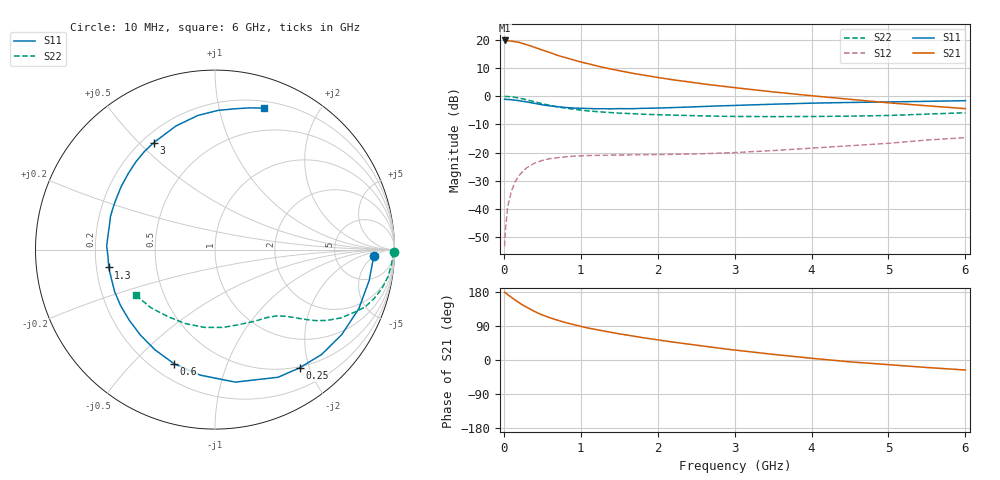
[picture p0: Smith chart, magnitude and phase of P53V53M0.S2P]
! SIEMENS Small Signal Semiconductors
! BFP183
! Si NPN RF Bipolar Junction Transistor in SOT143
! VCE = 3.5 V  IC = 3 mA
! Common Emitter S-Parameters:  March  1996
# GHz  S  MA  R  50
!  f  S11  S21  S12  S22
! GHz  MAG  ANG  MAG  ANG  MAG  ANG  MAG  ANG
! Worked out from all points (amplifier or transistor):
!   36 points, 10 MHz to 6 GHz, reference 50 ohm
!   highest |S21| = 19.8 dB at 10 MHz (marker M1)
!   |S21| within 3 dB of that: start of sweep to 458.7 MHz
!   unconditionally stable (mu >= 1): 1.886 GHz to 5.691 GHz
!   at 250 MHz: K = 0.15, MSG = 22.6 dB, |S12| = -26.5 dB
!   at 1.4 GHz: K = 0.78, MSG = 15.2 dB, |S12| = -20.9 dB
!   at 6 GHz: K = 0.94, MSG = 5.1 dB, |S12| = -14.7 dB
!   lowest NFmin = 1.10 dB at 450 MHz
!   S11 on the Smith chart (normalised r, x): 10 MHz: 15, -5; 250 MHz: 0.48, -1.85; 600 MHz: 0.28, -0.67; 1.3 GHz: 0.25, -0.08; 3 GHz: 0.25, +0.55; 6 GHz: 0.26, +1.37
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0.01  0.8851 -2.3  9.742 178.7  0.0022 87.7  0.9971 -0.9
0.02  0.8808 -4.7  9.661 177.6  0.0041 85.4  0.9912 -1.8
0.05  0.876 -11.4  9.675 172.5  0.011 85.8  0.9877 -4.5
0.1  0.8662 -22.4  9.489 165.2  0.0211 76.7  0.9754 -9.0
0.2  0.8333 -44.5  9.006 151.0  0.0396 66.3  0.9275 -17.1
0.25  0.8101 -54.4  8.581 144.5  0.0474 61.1  0.8958 -20.8
0.3  0.7933 -63.7  8.179 139.1  0.0543 56.6  0.8602 -23.6
0.4  0.7469 -81.3  7.366 128.0  0.0652 49.0  0.798 -28.5
0.5  0.7043 -96.7  6.585 118.8  0.0728 42.1  0.7384 -32.3
0.6  0.6757 -109.7  5.951 111.4  0.0783 37.2  0.6883 -35.1
0.7  0.6509 -120.9  5.292 104.9  0.0815 33.4  0.6476 -37.1
0.8  0.6321 -131.1  4.84 98.9  0.0843 30.2  0.6166 -38.7
0.9  0.6191 -140.5  4.422 93.8  0.0869 27.7  0.59 -40.1
1.1  0.6062 -157.3  3.756 84.1  0.0888 23.9  0.5488 -42.7
1.3  0.6005 -170.5  3.226 76.5  0.0901 21.3  0.5223 -45.1
1.8  0.6106 162.5  2.392 59.1  0.0919 19.3  0.4809 -51.5
2.2  0.6296 146.3  1.954 47.3  0.0932 19.6  0.4631 -57.7
3  0.6868 119.8  1.42 26.3  0.1003 22.9  0.4381 -73.2
3.5  0.7223 107.5  1.194 14.9  0.1089 24.7  0.4359 -84.3
4.5  0.7759 88.7  0.882 -4.9  0.1326 25.4  0.4437 -111.6
5.5  0.8127 76.3  0.677 -19.8  0.1674 23.1  0.4821 -137.8
6  0.8342 70.9  0.603 -26.4  0.1844 19.4  0.5097 -150.2
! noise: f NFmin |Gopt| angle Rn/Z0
0.45  1.1  0.37  35  0.3
0.9  1.15  0.34  85  0.23
1.8  1.9  0.35  160  0.13
